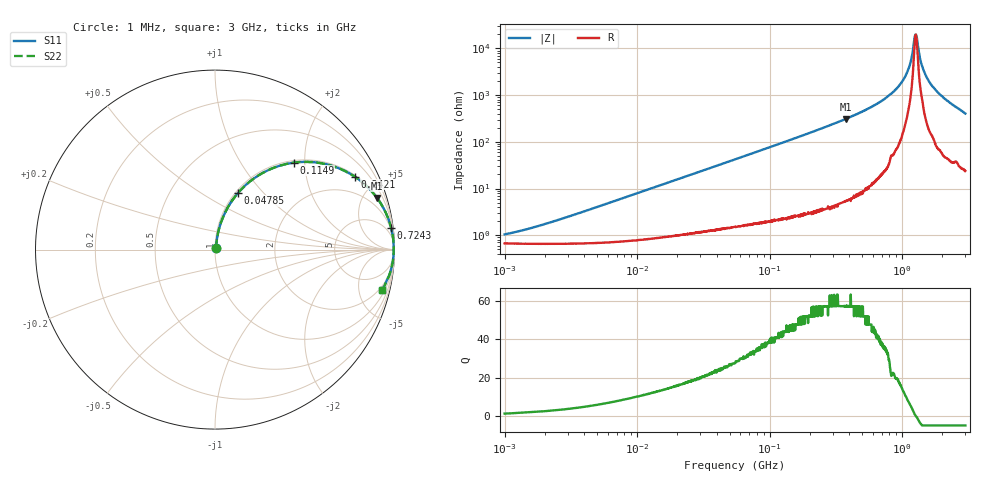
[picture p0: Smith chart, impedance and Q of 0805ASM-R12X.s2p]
!s-Parameter Generated by FASTRON Sdn. Bhd.
!FASTRON P/N : 0805ASM-R12X
!Keysight Technologies: E4991B_MY54100416_A.01.15
!Date: Fri Jun 19 14:50:18 2026
!Version  :Rev00  Fri Jun 19 14:50:18 2026
!Data & Calibration Information:
!Freq  S11  S21  S12  S22
!PortZ  Port1:50+j0  Port2:50+j0
!When reading reference impedance value at option line is always used.
! Remarks : This data is being provided solely for informational purposes.
# Hz S dB R 50
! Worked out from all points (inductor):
!   1601 points, 1 MHz to 3 GHz, reference 50 ohm
!   read as one part in series: L = 127 nH near 2.474 MHz
!   highest Q = 57.4 at 377.9 MHz (marker M1), where L = 131 nH
!   self-resonance near 1.262 GHz
!   S11 on the Smith chart (normalised r, x): 1 MHz: 1.01, +0.02; 47.85 MHz: 1.03, +0.74; 114.9 MHz: 1.04, +1.76; 242.1 MHz: 1.07, +3.79; 724.3 MHz: 1, +16; 3 GHz: 1.48, -8.06
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1000000  -39.70 49.6  -0.06 -0.5  -0.06 -0.5  -39.70 49.6
3804036  -30.20 75.9  -0.06 -1.7  -0.06 -1.7  -30.20 75.9
1.447069e7  -19.00 79.2  -0.13 -6.4  -0.13 -6.4  -19.00 79.2
4.785025e7  -9.33 67.8  -0.66 -19.9  -0.66 -19.9  -9.33 67.8
5.504702e7  -8.30 65.3  -0.82 -22.6  -0.82 -22.6  -8.30 65.3
1.148668e8  -3.70 47.9  -2.59 -40.7  -2.59 -40.7  -3.70 47.9
2.083556e8  -1.48 31.4  -5.66 -57.5  -5.66 -57.5  -1.48 31.4
2.421036e8  -1.13 27.6  -6.69 -61.4  -6.69 -61.4  -1.13 27.6
3.779341e8  -0.47 17.7  -10.30 -71.3  -10.30 -71.3  -0.47 17.7
7.243229e8  -0.10 7.1  -18.20 -81.3  -18.20 -81.3  -0.10 7.1
7.925923e8  -0.07 5.8  -19.90 -82.2  -19.90 -82.2  -0.07 5.8
9.395906e8  -0.05 3.7  -23.80 -83.1  -23.80 -83.1  -0.05 3.7
1.064802e9  -0.04 2.1  -28.50 -82.3  -28.50 -82.3  -0.04 2.1
1.142072e9  -0.03 1.3  -32.90 -79.5  -32.90 -79.5  -0.03 1.3
1.231095e9  -0.04 0.3  -43.40 -51.8  -43.40 -51.8  -0.04 0.3
1.268618e9  -0.04 -0.0  -46.00 3.3  -46.00 3.3  -0.04 -0.0
1.300759e9  -0.04 -0.3  -43.30 47.4  -43.30 47.4  -0.04 -0.3
1.374365e9  -0.04 -1.0  -34.90 74.8  -34.90 74.8  -0.04 -1.0
1.423359e9  -0.04 -1.4  -32.00 78.2  -32.00 78.2  -0.04 -1.4
1.637435e9  -0.06 -3.2  -24.90 81.8  -24.90 81.8  -0.06 -3.2
2.102926e9  -0.12 -6.8  -18.50 80.0  -18.50 80.0  -0.12 -6.8
3e9  -0.38 -13.7  -12.50 72.9  -12.50 72.9  -0.38 -13.7
